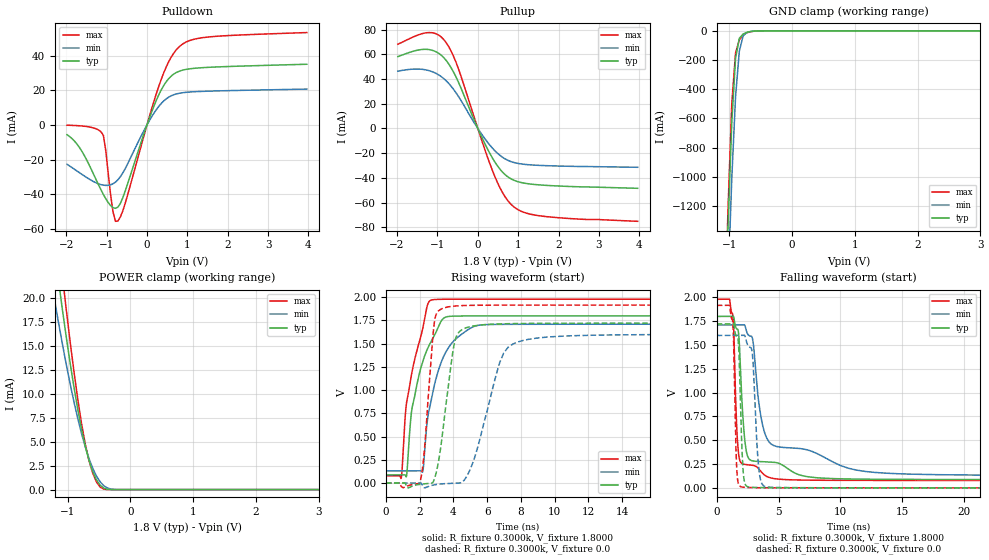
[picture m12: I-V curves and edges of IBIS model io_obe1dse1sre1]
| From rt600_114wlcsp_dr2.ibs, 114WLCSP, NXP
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[Model] io_obe1dse1sre1
|   Model io_obe1dse1sre1
| Library cells for typ/min/max conditions are connected as defined below:
|  pad - External Pad
|  ipp_do - Core Input
|  ipp_obe - Output Buffer Enable
|  REFH3V3 - vdd1v8
|  REFL3V3 - REFL3V3
|  gnde - gnde
|  ipp_dse - vdd
|  ipp_ina235_3v - NC
|  ipp_ina40_3v - NC
|  ipp_ina_mux - NC
|  ipp_ind - NC
|  ipp_ind_1p8v - NC
|  ipp_ind_3v - NC
|  ipp_sre - vdd
|  vdd - vdd
|  vdd1v8 - vdd1v8
|  vdda - vdde3v3
|  vdde3v3 - vdde3v3
| All other pins connected to ground
Model_type I/O
Polarity   Non-Inverting
Enable   Active-High
Vinl =   0.5400V
Vinh =   1.2600V
Vmeas =  0.9000V
Cref =   25.0000pF
Rref =   0.5000k
Vref =   0.0V
C_comp   2.2456pF   2.1702pF   2.3895pF
[Temperature Range]   25.0000   0.1250k   -40.0000
[Voltage Range]   1.8000V   1.7100V   1.9800V
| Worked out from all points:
|   slope of the pulldown table from 0 to 0.27 V, typ, clamps not added: 16.6 ohm
|   slope of the pullup table from 0 to 0.27 V, typ, clamps not added: 14.6 ohm
|   GND clamp passes 1 mA (typ) near -0.57 V on its own axis
|   POWER clamp passes 1 mA (typ) near -0.54 V on its own axis
|   rising waveform, R_fixture 0.3000k, V_fixture 1.8000: 20-80 % time 1.13ns typ, 1.17ns min, 1.05ns max; typ from 0.087 V to 1.8 V
|   rising waveform, R_fixture 0.3000k, V_fixture 0.0: 20-80 % time 720ps typ, 1.38ns min, 467ps max; typ from 0 V to 1.72 V
|   falling waveform, R_fixture 0.3000k, V_fixture 1.8000: 20-80 % time 485ps typ, 1.54ns min, 306ps max; typ from 1.8 V to 0.087 V
|   falling waveform, R_fixture 0.3000k, V_fixture 0.0: 20-80 % time 253ps typ, 369ps min, 195ps max; typ from 1.72 V to 0 V
[Pulldown]
|Voltage   I(typ)   I(min)   I(max)
-1.98V    -5.65mA    -22.75mA   -160uA
-1.62V    -14.97mA   -28.49mA   -590uA
-1.08V    -40.24mA   -34.85mA   -6.067mA
-840mV    -47.89mA   -34.01mA   -50.49mA
-780mV    -48.24mA   -33.06mA   -55.75mA
-720mV    -47.53mA   -31.71mA   -55.6mA
-540mV    -38.27mA   -25.32mA   -45.39mA
240mV     14.7mA     9.107mA    18.7mA
540mV     26.85mA    16.1mA     36.66mA
780mV     30.9mA     18.23mA    44.81mA
1.44V     33.22mA    19.47mA    50.67mA
3.96V     35.11mA    20.73mA    53.44mA
[Pullup]
|Voltage   I(typ)   I(min)   I(max)
-1.98V    58.06mA    46.32mA    68.12mA
-1.2V     63.76mA    46.68mA    77.56mA
-960mV    60.59mA    43.12mA    75.31mA
-780mV    54.85mA    38.42mA    69.22mA
-480mV    37.43mA    25.91mA    48.3mA
60mV      -4.38mA    -2.967mA   -5.982mA
420mV     -27.07mA   -17.98mA   -38.74mA
660mV     -36.95mA   -24.37mA   -54.58mA
900mV     -42.07mA   -27.66mA   -63.71mA
1.2V      -44.59mA   -29.25mA   -68.57mA
1.68V     -46.09mA   -30.15mA   -71.35mA
3.96V     -48.5mA    -31.49mA   -75.21mA
[GND_clamp]
|Voltage   I(typ)   I(min)   I(max)
-1.98V    -17.57A    -17.55A    -18.13A
-1.08V    -2.185A    -2.567A    -2.121A
-1.02V    -1.339A    -1.74A     -1.223A
-960mV    -630.1mA   -1.012A    -499.4mA
-900mV    -189.5mA   -452.2mA   -152mA
-840mV    -51.34mA   -139.9mA   -62.86mA
-780mV    -22.28mA   -35.54mA   -26.58mA
-720mV    -10.62mA   -11.15mA   -13.18mA
-600mV    -1.527mA   -2.152mA   -2.249mA
-480mV    -85.63uA   -243.9uA   -63.17uA
3.96V     0A         0A         0A
[POWER_clamp]
|Voltage   I(typ)   I(min)   I(max)
-1.98V    66.18mA    51.42mA    77.85mA
-1.26V    27.66mA    21.8mA     33.09mA
-1.2V     24.56mA    19.48mA    29.34mA
-1.14V    21.54mA    17.24mA    25.67mA
-1.08V    18.63mA    15.07mA    22.11mA
-1.02V    15.84mA    13mA       18.69mA
-840mV    8.434mA    7.464mA    9.5mA
-720mV    4.556mA    4.476mA    4.785mA
-600mV    1.876mA    2.218mA    1.703mA
-540mV    1.008mA    1.402mA    786.9uA
-420mV    135uA      383.7uA    43.39uA
3.96V     0A         0A         0A
[Ramp]
| variable   typ   min   max
dV/dt_r  0.8235/1.4240n   0.6782/3.0009n   0.9804/0.8173n
dV/dt_f  0.7767/6.4045n   0.5489/11.2396n   0.9301/3.1390n
R_load = 50.0000
[Rising Waveform]
R_fixture= 0.3000k
V_fixture= 1.8000
V_fixture_min= 1.7100
V_fixture_max= 1.9800
|time   V(typ)   V(min)   V(max)
0s        87.44mV    130.7mV    78.02mV
910.4ps   87.44mV    130.7mV    54.54mV
1.216ns   70.9mV     130.7mV    853.7mV
1.532ns   783.4mV    130.7mV    1.18V
2.175ns   1.303V     118.3mV    1.655V
2.501ns   1.459V     729.4mV    1.934V
3.146ns   1.695V     1.232V     1.978V
4.865ns   1.799V     1.651V     1.98V
7.013ns   1.8V       1.709V     1.98V
500ns     1.8V       1.71V      1.98V
[Rising Waveform]
R_fixture= 0.3000k
V_fixture= 0.0
V_fixture_min= 0.0
V_fixture_max= 0.0
|time   V(typ)   V(min)   V(max)
0s        22.64nV    701nV      38.04nV
2.034ns   -13.06mV   589.4uV    19.3mV
2.292ns   -7.877mV   -51.04mV   369.5mV
2.804ns   13.31mV    -21.31mV   1.616V
3.057ns   171.9mV    -13.67mV   1.841V
4.082ns   1.521V     -1.819mV   1.905V
4.956ns   1.682V     130.1mV    1.913V
7.242ns   1.716V     1.461V     1.916V
12.3ns    1.721V     1.592V     1.916V
500ns     1.721V     1.6V       1.916V
[Falling Waveform]
R_fixture= 0.3000k
V_fixture= 1.8000
V_fixture_min= 1.7100
V_fixture_max= 1.9800
|time   V(typ)   V(min)   V(max)
0s        1.8V       1.71V      1.98V
1.296ns   1.8V       1.71V      1.818V
1.634ns   1.668V     1.71V      592mV
1.898ns   1.325V     1.71V      277.6mV
2.182ns   627.9mV    1.711V     247.9mV
2.524ns   323.7mV    1.611V     241.9mV
3.962ns   273.4mV    547.8mV    125.8mV
6.068ns   173.8mV    418.9mV    84.13mV
22.23ns   87.58mV    133.6mV    78.02mV
500ns     87.44mV    130.7mV    78.02mV
[Falling Waveform]
R_fixture= 0.3000k
V_fixture= 0.0
V_fixture_min= 0.0
V_fixture_max= 0.0
|time   V(typ)   V(min)   V(max)
0s        1.721V     1.6V       1.916V
1.289ns   1.721V     1.6V       1.748V
1.56ns    1.598V     1.6V       394.6mV
1.712ns   1.569V     1.6V       67.3mV
2.15ns    153.1mV    1.6V       6.915mV
2.745ns   6.394mV    1.472V     2.526mV
2.923ns   5.045mV    1.35V      1.94mV
3.475ns   3.054mV    127.9mV    1.016mV
4.65ns    1.241mV    4.908mV    499uV
500ns     389.7nV    1.16uV     255nV
